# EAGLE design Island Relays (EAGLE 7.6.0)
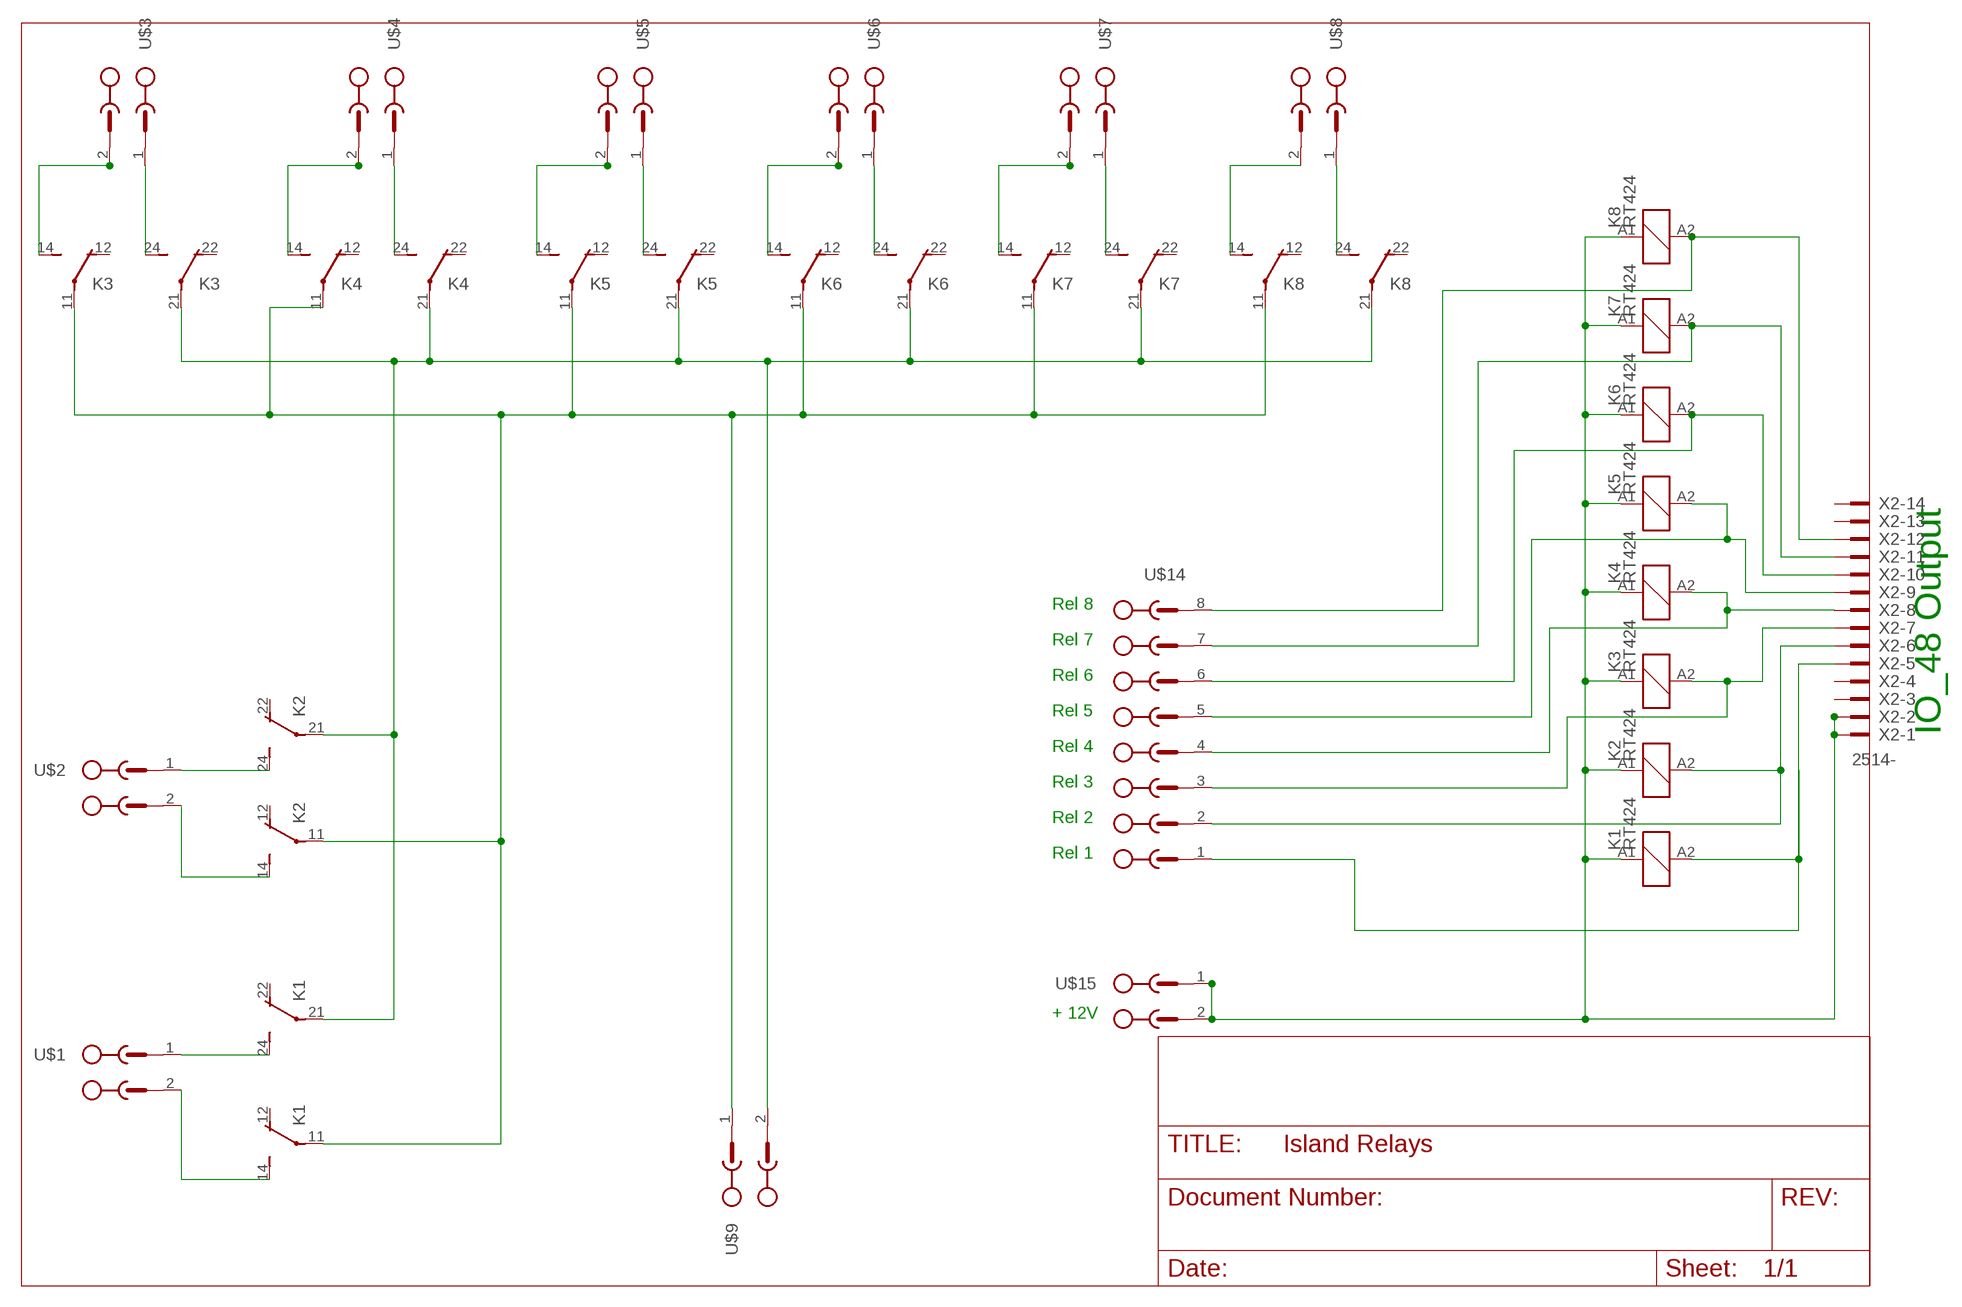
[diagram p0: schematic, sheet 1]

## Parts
K1  RT424  [RT2C/O]
K2  RT424  [RT2C/O]
K3  RT424  [RT2C/O]
K4  RT424  [RT2C/O]
K5  RT424  [RT2C/O]
K6  RT424  [RT2C/O]
K7  RT424  [RT2C/O]
K8  RT424  [RT2C/O]
U$1  PT1_5_2-PVH-50  [PT1_5_2-PVH-50]
U$2  PT1_5_2-PVH-50  [PT1_5_2-PVH-50]
U$3  PT1_5_2-PVH-50  [PT1_5_2-PVH-50]
U$4  PT1_5_2-PVH-50  [PT1_5_2-PVH-50]
U$5  PT1_5_2-PVH-50  [PT1_5_2-PVH-50]
U$6  PT1_5_2-PVH-50  [PT1_5_2-PVH-50]
U$7  PT1_5_2-PVH-50  [PT1_5_2-PVH-50]
U$8  PT1_5_2-PVH-50  [PT1_5_2-PVH-50]
U$9  PT1_5_2-PVH-50  [PT1_5_2-PVH-50]
U$14  PT1_5_8-PVH-50  [PT1_5_8-PVH-50]
U$15  PT1_5_2-PVH-50  [PT1_5_2-PVH-50]
X2  2514-  [PAK100/2500-14]

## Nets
N$1 [Track]: K1.14(2:S) U$1.2(SK1)
N$2 [Track]: K1.24(3:S) U$1.1(SK)
N$3 [Track]: K2.14(2:S) U$2.2(SK1)
N$4 [Track]: K2.24(3:S) U$2.1(SK)
N$5 [Track]: K3.14(2:S) U$3.2(SK1)
N$6 [Track]: K3.24(3:S) U$3.1(SK)
N$7 [Track]: K4.14(2:S) U$4.2(SK1)
N$8 [Track]: K4.24(3:S) U$4.1(SK)
N$9 [Track]: K5.14(2:S) U$5.2(SK1)
N$10 [Track]: K5.24(3:S) U$5.1(SK)
N$11 [Track]: K6.14(2:S) U$6.2(SK1)
N$12 [Track]: K6.24(3:S) U$6.1(SK)
N$13 [Track]: K7.14(2:S) U$7.2(SK1)
N$14 [Track]: K7.24(3:S) U$7.1(SK)
N$15 [Track]: K8.14(2:S) U$8.2(SK1)
N$16 [Track]: K8.24(3:S) U$8.1(SK)
N$17 [Track]: K1.A1 K2.A1 K3.A1 K4.A1 K5.A1 K6.A1 K7.A1 K8.A1 U$15.1(SK) U$15.2(SK1) X2.1 X2.2
N$18 [Track]: K1.21(3:P) K2.21(3:P) K3.21(3:P) K4.21(3:P) K5.21(3:P) K6.21(3:P) K7.21(3:P) K8.21(3:P) U$9.2(SK1)
N$19: K2.A2 U$14.2(SK1) X2.6
N$20 [Track]: K1.11(2:P) K2.11(2:P) K3.11(2:P) K4.11(2:P) K5.11(2:P) K6.11(2:P) K7.11(2:P) K8.11(2:P) U$9.1(SK)
N$21: K6.A2 U$14.6(SK5) X2.10
N$22: K7.A2 U$14.7(SK6) X2.11
N$23: K4.A2 U$14.4(SK3) X2.8
N$24: K5.A2 U$14.5(SK4) X2.9
N$25: K8.A2 U$14.8(SK7) X2.12
N$28: K3.A2 U$14.3(SK2) X2.7
N$30: K1.A2 U$14.1(SK) X2.5
Unconnected: K1.12(2:O) K1.22(3:O) K2.12(2:O) K2.22(3:O) K3.12(2:O) K3.22(3:O) K4.12(2:O) K4.22(3:O) K5.12(2:O) K5.22(3:O) K6.12(2:O) K6.22(3:O) K7.12(2:O) K7.22(3:O) K8.12(2:O) K8.22(3:O) X2.3 X2.4 X2.13 X2.14

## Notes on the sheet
- Rel 8
- Rel 7
- Rel 6
- Rel 5
- IO_48 Output
- Rel 4
- Rel 3
- Rel 2
- Rel 1
- + 12V

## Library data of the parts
K1-K8 = BDL-Boards:RT42?*: Power PCB Relay SCHRACK 2 pole 8 A, DC and AC-coil Source: http://www.schrack.com/.. 5842.pdf
U$1-U$9 U$15 = BDL-Boards:PT1_5_2-PVH-50
U$14 = BDL-Boards:PT1_5_8-PVH-50
X2 = con-3m:2514-: 3M (TM) Pak 100 4-Wall Header Source: 3M; OC_FARNELL: unknown; OC_NEWARK: unknown

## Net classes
0 default: width 0.762 mm, drill 0.508 mm, clearance 0.381 mm
1 GND: width 0.762 mm, drill 0.508 mm, clearance 0.381 mm
2 VCC1: width 1.27 mm, drill 0.508 mm, clearance 0.381 mm
3 VCC2: width 0.762 mm, drill 0.508 mm, clearance 0.381 mm
4 Track: width 2.032 mm, drill 0.508 mm, clearance 0.381 mm

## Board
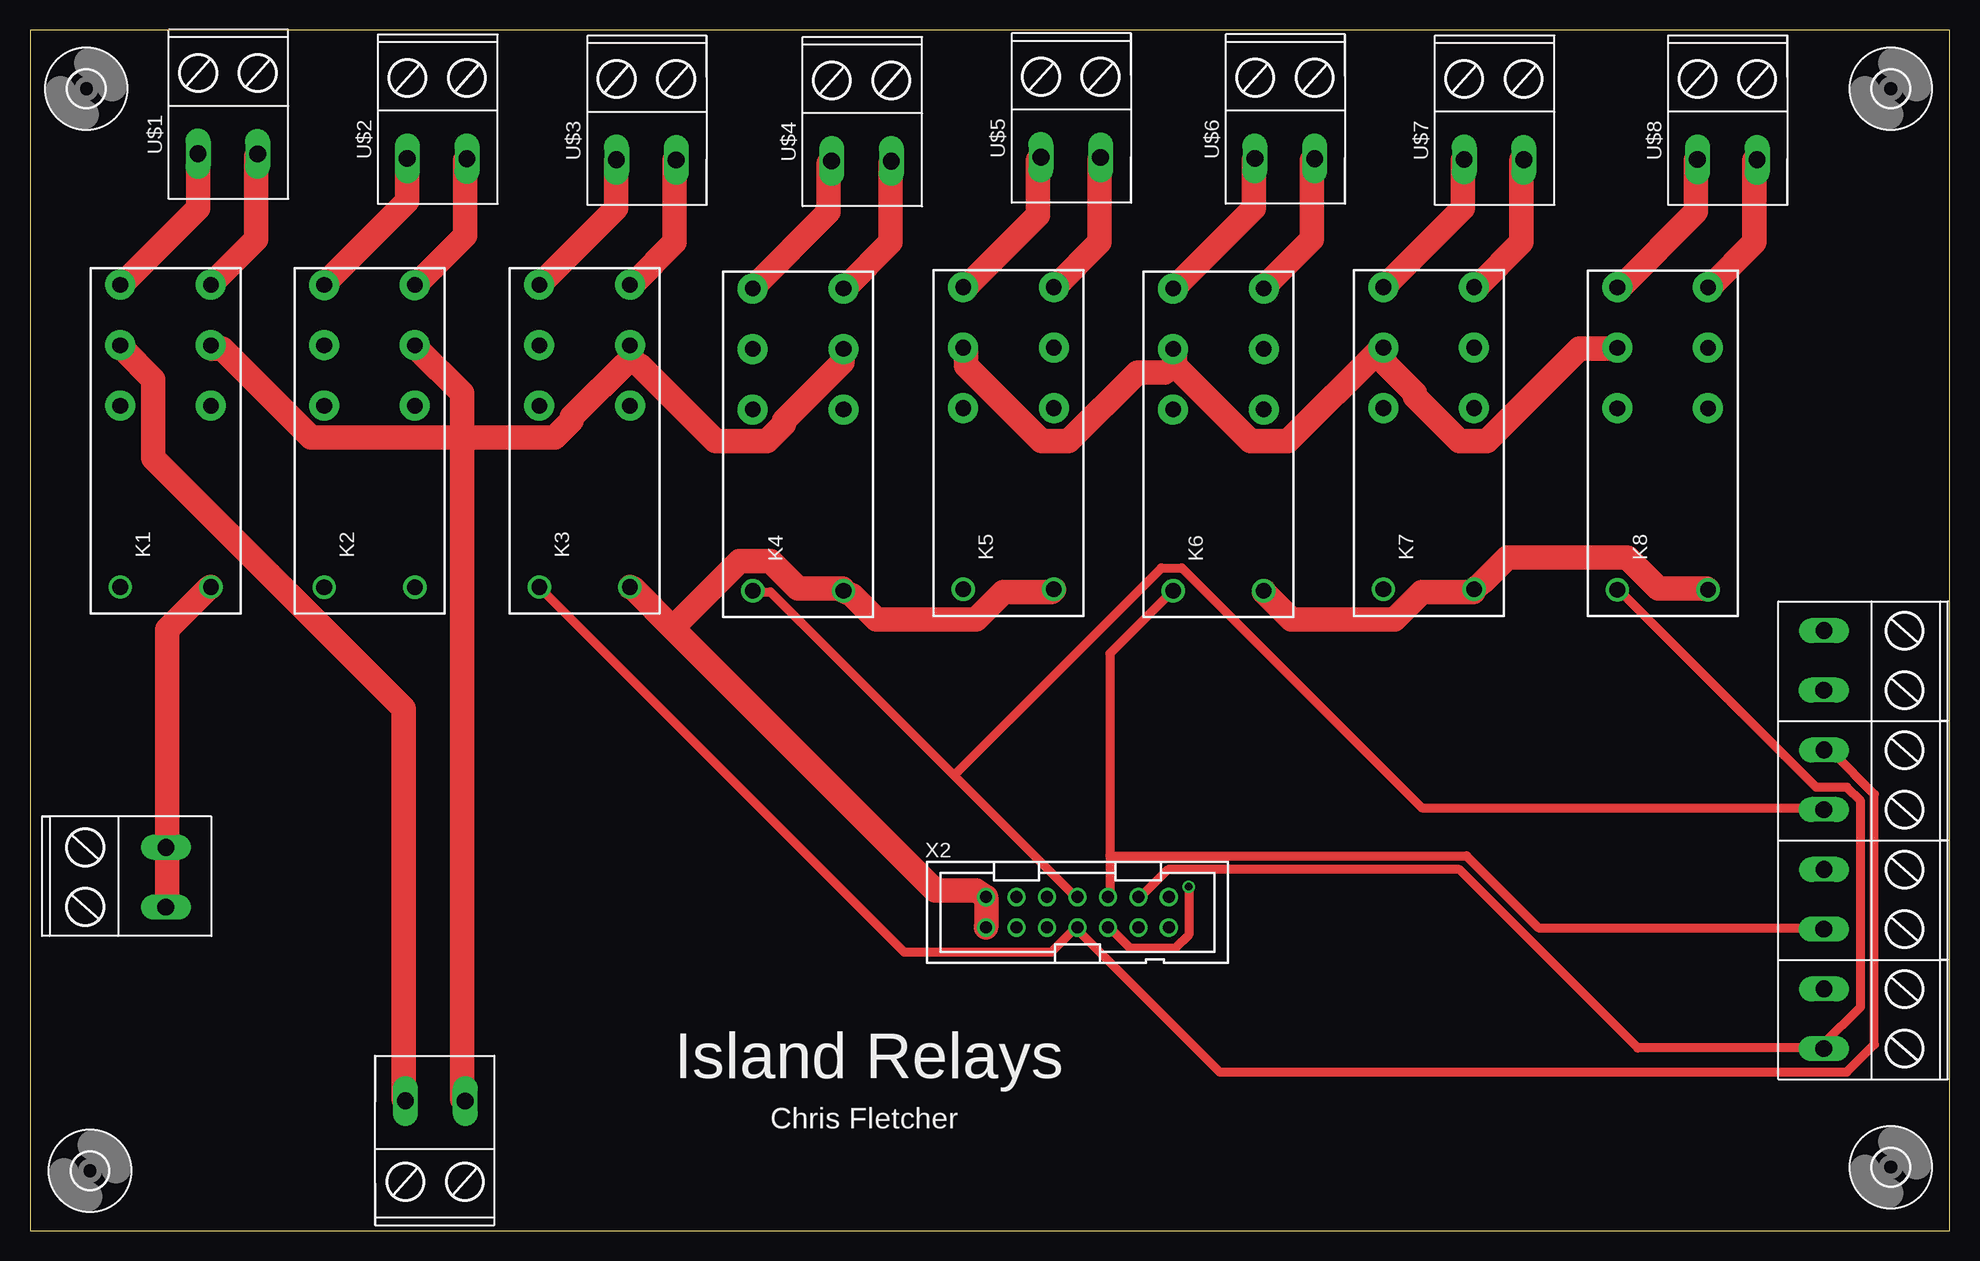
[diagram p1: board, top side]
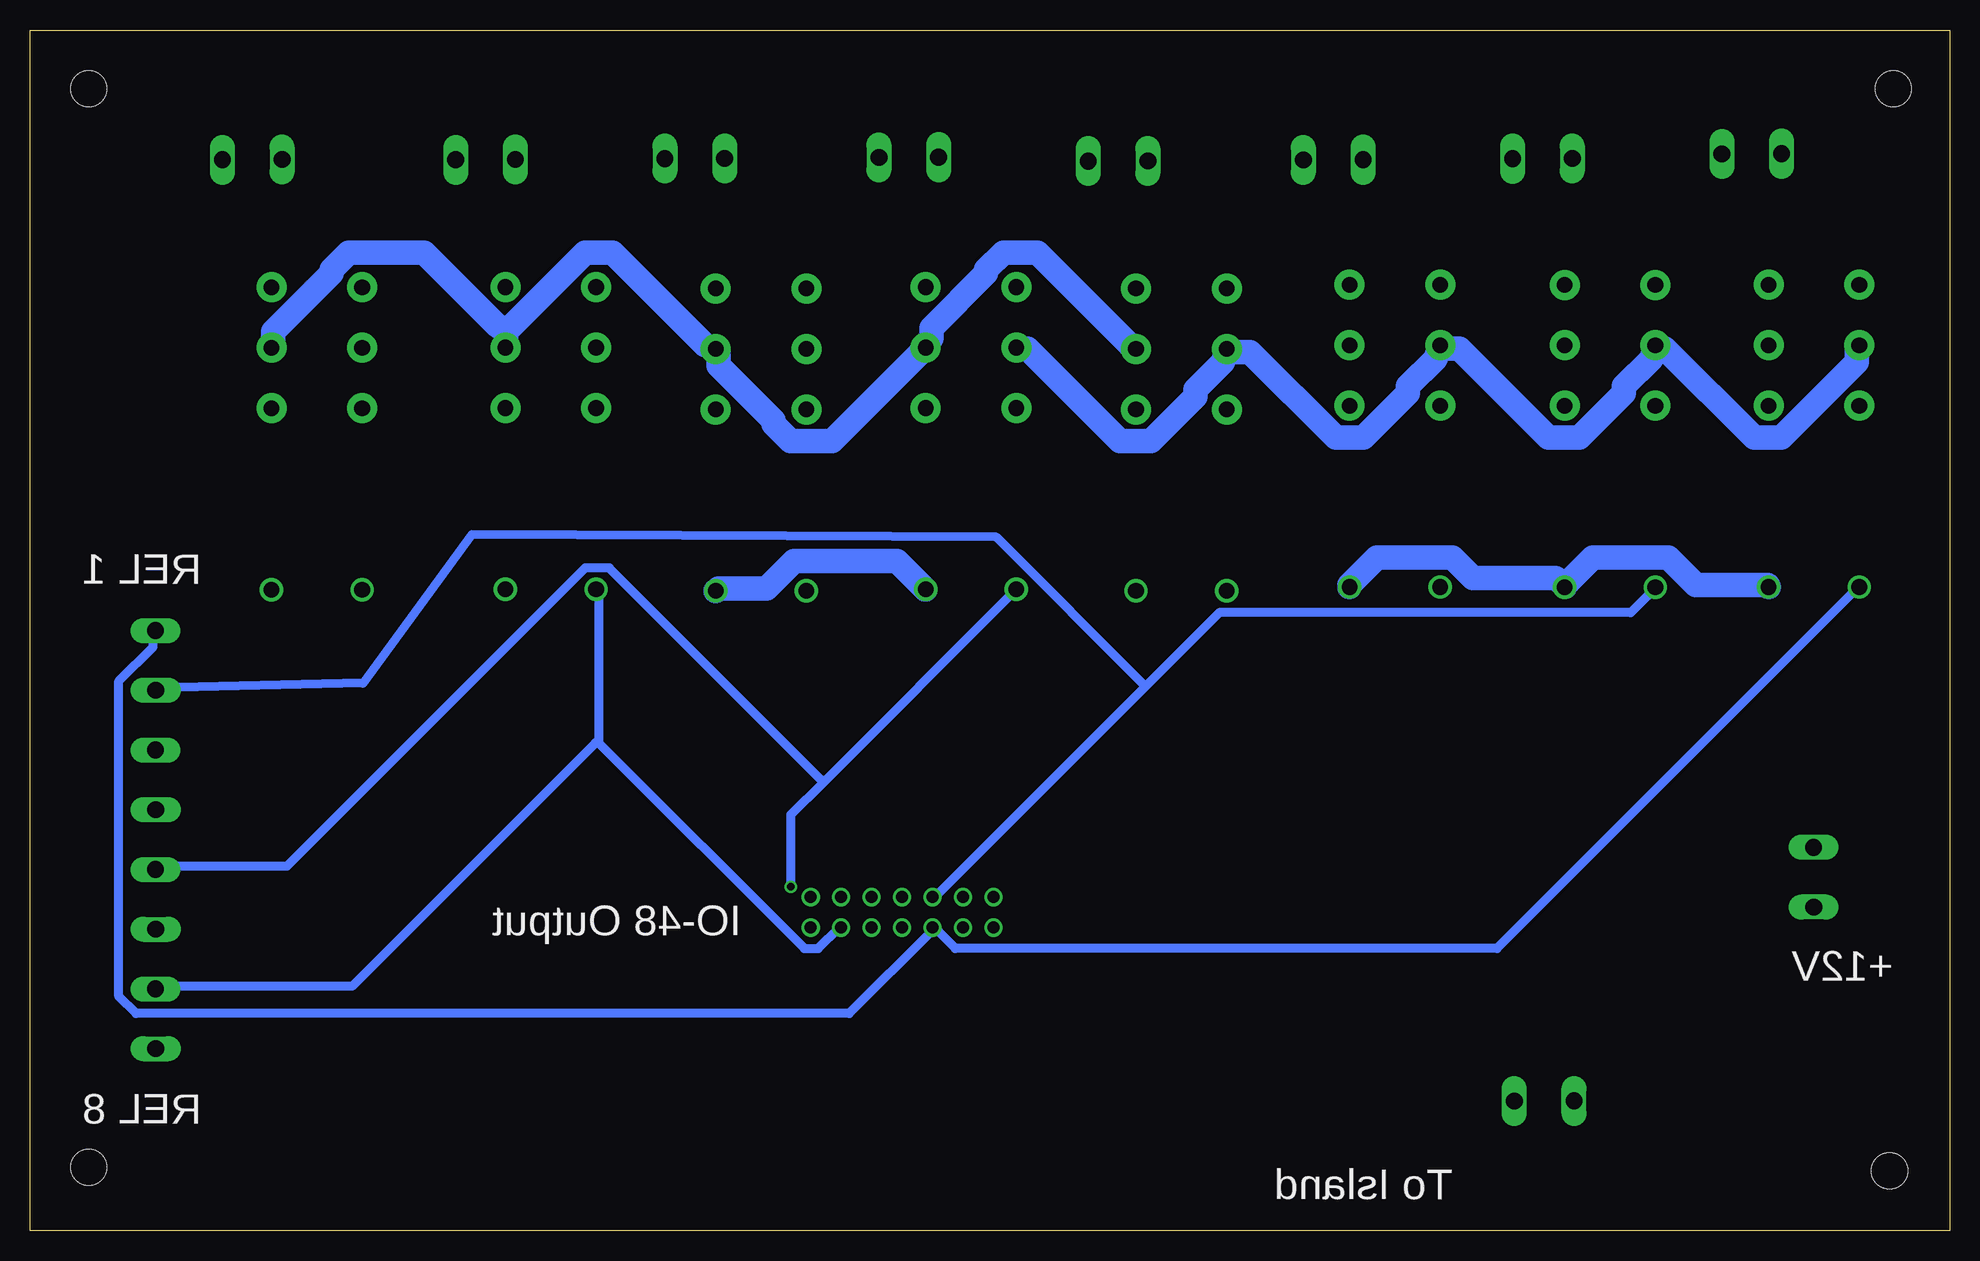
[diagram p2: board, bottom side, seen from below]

Size 160 x 100.1 mm. Coordinates in mm from the lower left corner, seen from the top.
Outline: 0,0 160,0 160,100.1 0,100.1 0,0
Copper layers (1*16): Top 0.035mm / dielectric 1.5mm / Bottom 0.035mm
Design rules "default": minimum track width 10mil, minimum drill 24mil, track to track 8mil, track to pad 8mil, pad to pad 8mil, via to via 8mil, smd to smd 8mil, copper to edge 40mil, drill to drill 8mil, minimum pad ring 10mil, minimum via ring 8mil, stop-mask expansion 4mil, vias tented up to drill 0mil, thermal gap 10mil

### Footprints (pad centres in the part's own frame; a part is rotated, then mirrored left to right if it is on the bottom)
RT2C/O = drill 1.3 pad 2.5: 11 7.56,-3.68; 12 2.52,-3.68; 14 12.6,-3.68; 21 7.56,3.88; 22 2.52,3.88; 24 12.6,3.88 | drill 1.3: A1 -12.6,-3.68; A2 -12.6,3.88
PT1_5_2-PVH-50 = drill 1.397 long: 1 1.917,2.42; 2 -3.059,2.44
3,0 = hole 3: 0,0
PT1_5_8-PVH-50 = drill 1.397 long: 1 22.238,4.96; 2 17.261,4.98; 3 12.277,4.96; 4 7.301,4.98; 5 2.317,4.96; 6 -2.659,4.98; 7 -7.643,4.96; 8 -12.619,4.98
PAK100/2500-14 = drill 1 pad 1.422: 1 -7.62,-1.27; 2 -7.62,1.27; 3 -5.08,-1.27; 4 -5.08,1.27; 5 -2.54,-1.27; 6 -2.54,1.27; 7 0,-1.27; 8 0,1.27; 9 2.54,-1.27; 10 2.54,1.27; 11 5.08,-1.27; 12 5.08,1.27; 13 7.62,-1.27; 14 7.62,1.27

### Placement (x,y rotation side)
K1  11.4,66.26 90 top
K2  28.4,66.25 90 top
K3  46.33,66.26 90 top
K4  64.13,65.95 90 top
K5  81.66,66.06 90 top
K6  99.16,65.95 90 top
K7  116.69,66.06 90 top
K8  136.19,66.05 90 top
U$1  15.92,92.21 180 top
U$2  33.36,91.81 180 top
U$3  50.8,91.71 180 top
U$4  68.74,91.61 180 top
U$5  86.18,91.91 180 top
U$6  104.02,91.82 180 top
U$7  121.46,91.72 180 top
U$8  140.9,91.72 180 top
U$9  34.36,8.38 0 top
U$10  [3,0]  4.7,95.2 0 top
U$11  [3,0]  5,5 0 top
U$12  [3,0]  155.1,95.2 0 top
U$13  [3,0]  155.1,5.3 0 top
U$14  154.5,27.8 90 top
U$15  8.9,28.9 270 top
X2  87.3,26.54 0 top

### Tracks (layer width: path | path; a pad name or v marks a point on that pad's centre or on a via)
N$1
  Top 2.032: U$1.2 18.86,89.54 18.86,82.68 15.14,78.97 K1.14
N$2
  Top 2.032: U$1.1 14,89.54 14,85.25 7.71,78.97 K1.24
N$3
  Top 2.032: U$2.2 36.29,89.25 36.29,82.97 32.29,78.97 K2.14
N$4
  Top 2.032: U$2.1 31.43,89.25 31.43,85.82 24.57,78.97 K2.24
N$5
  Top 2.032: U$3.2 53.72,89.25 53.72,82.4 50.29,78.97 K3.14
N$6
  Top 2.032: U$3.1 48.86,89.25 48.86,85.25 42.58,78.97 K3.24
N$7
  Top 2.032: U$4.2 71.72,88.97 71.72,82.4 68.01,78.68 K4.14
N$8
  Top 2.032: U$4.1 66.58,88.97 66.58,84.97 60.29,78.68 K4.24
N$9
  Top 2.032: U$5.2 89.15,89.25 89.15,82.4 85.44,78.68 K5.14
N$10
  Top 2.032: U$5.1 84.01,89.25 84.01,84.68 78.01,78.68 K5.24
N$11
  Top 2.032: U$6.2 106.87,89.25 106.87,82.68 102.87,78.68 K6.14
N$12
  Top 2.032: U$6.1 102.01,89.25 102.01,85.25 95.44,78.68 K6.24
N$13
  Top 2.032: U$7.2 124.3,89.25 124.3,82.4 120.59,78.68 K7.14
N$14
  Top 2.032: U$7.1 119.44,89.25 119.44,85.25 112.87,78.68 K7.24
N$15
  Top 2.032: U$8.2 143.73,89.25 143.73,82.4 140.02,78.68 K8.14
N$16
  Top 2.032: U$8.1 138.88,89.25 138.88,84.97 132.59,78.68 K8.24
N$17
  Top 2.032: X2.1 79.72,25.53 79.72,27.53 X2.2 78.87,28.39 75.44,28.39 53.58,50.25 | 53.58,50.25 50.29,53.54 K3.A1 | 53.58,50.25 59.15,55.82 61.72,55.82 64.01,53.54 67.72,53.54 K4.A1 68.58,52.96 70.58,50.96 78.87,50.96 81.15,53.25 85.15,53.25 K5.A1 | K6.A1 102.87,53.25 105.16,50.96 113.73,50.96 116.01,53.25 120.3,53.25 K7.A1 121.16,54.11 123.16,56.11 133.16,56.11 135.73,53.54 139.73,53.54 K8.A1 | U$15.1 11.43,27.25 11.43,31.82 U$15.2 11.43,32.96 11.43,50.11 14.86,53.54 K1.A1
  Bottom 2.032: 32,53.82 29.72,56.11 23.43,56.11 21.14,53.82 15.14,53.82 K1.A1 | 32,53.82 K2.A1 | K6.A1 102.58,53.54 98.58,53.54 96.3,55.82 87.72,55.82 85.44,53.54 K5.A1 | 32,53.82 32.86,54.39 39.72,54.39 41.43,56.11 47.72,56.11 50.01,53.82 K3.A1
N$18
  Top 2.032: 95.44,72.11 95.44,73.25 K6.21 | 95.44,72.11 101.73,65.82 104.87,65.82 112.58,73.54 K7.21 112.87,72.39 115.44,69.82 115.44,69.54 119.16,65.82 121.44,65.82 129.16,73.54 132.3,73.54 K8.21 | U$9.2 31.15,10.96 31.15,43.53 10.29,64.39 10.29,70.97 7.71,73.54 K1.21 | 95.44,72.11 94.58,71.54 92.3,71.54 86.58,65.82 84.3,65.82 78.01,72.11 78.01,73.54 K5.21
  Bottom 2.032: K1.21 7.71,73.54 7.71,72.39 14,66.11 16.29,66.11 23.72,73.54 24.29,73.54 K2.21 24.86,72.68 27.15,70.39 27.15,69.82 30.86,66.11 33.43,66.11 40.86,73.54 42.29,73.54 K3.21 42.86,72.68 45.15,70.39 45.15,69.82 48.86,66.11 51.15,66.11 58.29,73.25 60.01,73.25 K4.21 60.58,72.39 62.87,70.11 62.87,69.54 66.58,65.82 69.15,65.82 76.87,73.54 77.72,73.54 K5.21
N$19
  Bottom 0.762: 67.01,45.39 60.87,51.54 26.57,51.54 24.57,53.54 K2.A2 | 67.01,45.39 84.58,27.82 X2.6 | 67.01,45.39 79.44,57.82 123.17,58.02 132.24,45.65 149.45,45.25 U$14.2
N$20
  Top 2.032: 36.01,66.11 36.01,69.82 32.29,73.54 K2.11 | 36.01,66.11 36.01,10.96 U$9.1 | 36.01,66.11 23.43,66.11 16,73.54 15.14,73.54 K1.11 | 50.01,72.68 50.01,73.54 K3.11 | 50.01,72.68 45.15,67.82 45.15,67.54 43.72,66.11 36.01,66.11 | K4.11 67.72,73.25 67.72,72.39 62.87,67.54 62.87,67.25 61.44,65.82 57.15,65.82 50.86,72.11 50.01,72.68
  Bottom 2.032: 120.3,74.97 120.3,73.82 K7.11 | 120.3,74.97 113.73,81.54 111.44,81.54 103.73,73.82 K6.11 102.58,73.25 102.58,72.11 98.01,67.54 98.01,67.25 96.58,65.82 93.15,65.82 85.44,73.54 K5.11 84.87,74.39 84.87,75.25 80.3,79.82 80.3,80.11 78.87,81.54 76.01,81.54 68.01,73.54 K4.11 | K8.11 139.73,73.82 139.73,74.97 134.87,79.82 134.87,80.11 133.44,81.54 127.16,81.54 121.16,75.54 120.3,74.97
N$21
  Top 0.762: 90.01,31.25 90.01,48.11 95.16,53.25 K6.A2 | 90.01,31.25 90.01,27.82 X2.10 | 90.01,31.25 119.73,31.25 125.73,25.25 149.45,25.25 U$14.6
N$22
  Bottom 0.762: 112.58,40.68 95.44,23.53 94.3,23.53 92.58,25.25 X2.11 | 112.58,40.68 112.58,53.25 K7.A2 | U$14.7 149.45,20.39 133.16,20.39 112.87,40.68 112.58,40.68
N$23
  Top 0.762: 77.01,37.96 61.72,53.25 60.29,53.25 K4.A2 | 77.01,37.96 87.15,27.82 X2.8 | 77.01,37.96 94.3,55.25 96.01,55.25 116.01,35.25 149.45,35.25 U$14.4
N$24  (via drill 0.61)
  Top 0.762: v96.58,28.68 96.58,24.68 95.44,23.53 91.73,23.53 90.01,25.25 X2.9
  Bottom 0.762: v96.58,28.68 96.58,34.68 93.87,37.39 | 93.87,37.39 78.01,53.25 K5.A2 | 93.87,37.39 111.73,55.25 113.73,55.25 138.59,30.39 149.45,30.39 U$14.5
N$25
  Top 0.762: X2.12 92.58,27.82 94.87,30.1 119.16,30.1 134.02,15.24 149.45,15.24 U$14.8 149.45,15.53 152.59,18.67 152.59,35.82 151.45,36.96 148.88,36.96 132.59,53.25 K8.A2
N$28
  Top 0.762: K3.A2 42.58,53.54 72.87,23.25 85.15,23.25 87.15,25.25 X2.7 87.44,24.96 99.16,13.24 151.45,13.24 153.73,15.53 153.73,36.39 150.3,39.82 149.73,39.82 U$14.3
N$30
  Bottom 0.762: K1.A2 7.71,53.54 37.72,23.53 82.87,23.53 84.58,25.25 X2.5 84.87,24.96 91.73,18.1 151.16,18.1 152.59,19.53 152.59,45.82 149.73,48.68 149.73,49.82 U$14.1

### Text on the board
tPlace: Island Relays | Chris Fletcher
bPlace: REL 1 | IO-48 Output | +12V | REL 8 | To Island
